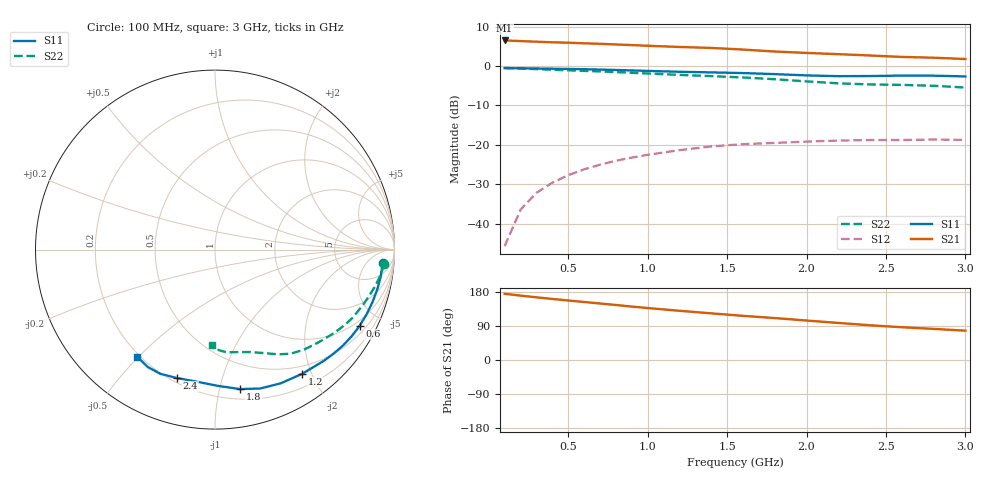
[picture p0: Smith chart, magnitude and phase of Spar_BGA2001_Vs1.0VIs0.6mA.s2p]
! Filename: 1G1.001
! Title: BGA2001 X0297-20 HFE=80
! Bias: Vce=1V,Ic=.6mA
! Company: NXP Semiconductors NL
! User: Quality&Reliability T&D
! Measure time: 23 Oct 1998 / 09:07:58
#  MHz  S  MA  R 50
! Freq  S11  S21  S12  S22  :
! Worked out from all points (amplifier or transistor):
!   20 points, 100 MHz to 3 GHz, reference 50 ohm
!   highest |S21| = 6.5 dB at 100 MHz (marker M1)
!   |S21| within 3 dB of that: start of sweep to 1.907 GHz
!   unconditionally stable (mu >= 1): start of sweep to 102.7 MHz
!   at 400 MHz: K = 0.20, MSG = 17.8 dB, |S12| = -29.6 dB
!   at 1.2 GHz: K = 0.34, MSG = 13.1 dB, |S12| = -21.4 dB
!   at 3 GHz: K = 0.93, MSG = 10.3 dB, |S12| = -18.7 dB
!   S11 on the Smith chart (normalised r, x): 100 MHz: 12, -15; 600 MHz: 0.78, -3.89; 1.2 GHz: 0.38, -1.86; 1.8 GHz: 0.28, -1.16; 2.4 GHz: 0.22, -0.72; 3 GHz: 0.19, -0.50
100  0.9373 -4.6  2.11 174.7  0.005179 53.7  0.9471 -4.9
200  0.9355 -9.3  2.073 169.9  0.01499 83.5  0.9315 -9.2
300  0.9307 -14.0  2.035 165.4  0.0246 80.0  0.914 -13.1
400  0.9245 -18.7  2 161.1  0.03306 76.5  0.897 -16.7
500  0.9182 -23.3  1.976 157.1  0.0412 73.4  0.882 -20.1
600  0.9108 -27.8  1.941 153.1  0.04883 70.4  0.8671 -23.4
700  0.9016 -32.3  1.914 149.1  0.05596 67.4  0.8541 -26.6
800  0.8914 -36.8  1.877 145.2  0.06282 64.4  0.8379 -29.8
900  0.8791 -41.2  1.844 141.0  0.06888 61.3  0.8209 -32.9
1000  0.8668 -45.7  1.807 137.2  0.07471 58.7  0.8041 -36.1
1200  0.8455 -54.9  1.745 129.9  0.08555 53.3  0.7716 -42.5
1400  0.8302 -63.8  1.696 123.1  0.09551 48.3  0.7446 -48.7
1600  0.8139 -72.0  1.618 116.5  0.102 44.0  0.7157 -54.2
1800  0.7893 -79.9  1.527 110.7  0.1058 40.8  0.68 -59.1
2000  0.7603 -88.4  1.465 104.2  0.11 36.3  0.6383 -64.6
2200  0.7431 -97.8  1.414 97.8  0.1133 31.8  0.6031 -71.2
2400  0.746 -106.5  1.36 91.7  0.1151 28.4  0.5836 -78.1
2600  0.7561 -113.7  1.304 86.4  0.1151 26.8  0.5758 -83.6
2800  0.7539 -119.7  1.274 82.0  0.1167 24.2  0.5613 -87.7
3000  0.7378 -126.0  1.227 77.5  0.1155 22.5  0.5327 -92.0
